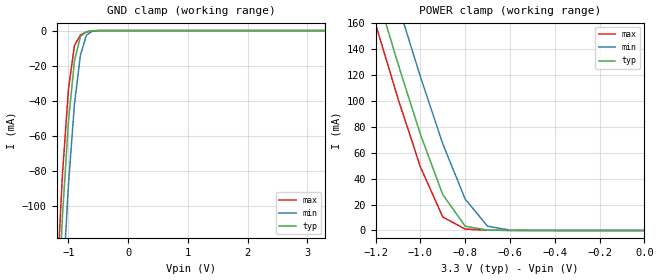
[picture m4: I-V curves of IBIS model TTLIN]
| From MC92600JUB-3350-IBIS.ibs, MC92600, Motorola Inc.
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|   Model TTLIN
[Model]   TTLIN
Model_type   Input
Vinl =   0.8000V
Vinh =   2.0000V
C_comp   7.0000pF   NA   NA
[Temperature Range]   40.0000   0.1050k   0.000
[Pullup Reference]   3.3000V   3.0000V   3.6000V
[Pulldown Reference]   0.000V   0.000V   0.000V
[POWER Clamp Reference]   3.3000V   3.0000V   3.6000V
[GND Clamp Reference]   0.000V   0.000V   0.000V
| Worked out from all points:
|   GND clamp passes 1 mA (typ) near -0.71 V on its own axis
|   POWER clamp passes 1 mA (typ) near -0.72 V on its own axis
[GND_clamp]
| voltage   I(typ)   I(min)   I(max)
-3.3V     -2.182A    -2.219A    -2.162A
-1.2V     -175.3mA   -221.5mA   -148.8mA
-1.1V     -105.2mA   -148.2mA   -81.3mA
-1V       -51.51mA   -87.49mA   -33.28mA
-900mV    -17.31mA   -41.89mA   -8.524mA
-800mV    -3.352mA   -14.01mA   -2.461mA
-700mV    -669.6uA   -2.594mA   -760.8uA
-600mV    -130.8uA   -311.5uA   -127.9uA
-500mV    -16.08uA   -47.06uA   -10.19uA
3.3V      1.715nA    860.2nA    117.7nA
[POWER_clamp]
| voltage   I(typ)   I(min)   I(max)
-3.3V     1.493A     1.532A     1.471A
-1.2V     186mA      232mA      159mA
-1.1V     128.5mA    174.2mA    101.7mA
-1V       74.15mA    118.5mA    48.99mA
-900mV    27.61mA    66.69mA    10.37mA
-800mV    3.292mA    24.21mA    1.065mA
-700mV    291.1uA    3.285mA    251.6uA
-600mV    49.84uA    254.8uA    43.21uA
0V        1.715nA    93.99nA    130nA
